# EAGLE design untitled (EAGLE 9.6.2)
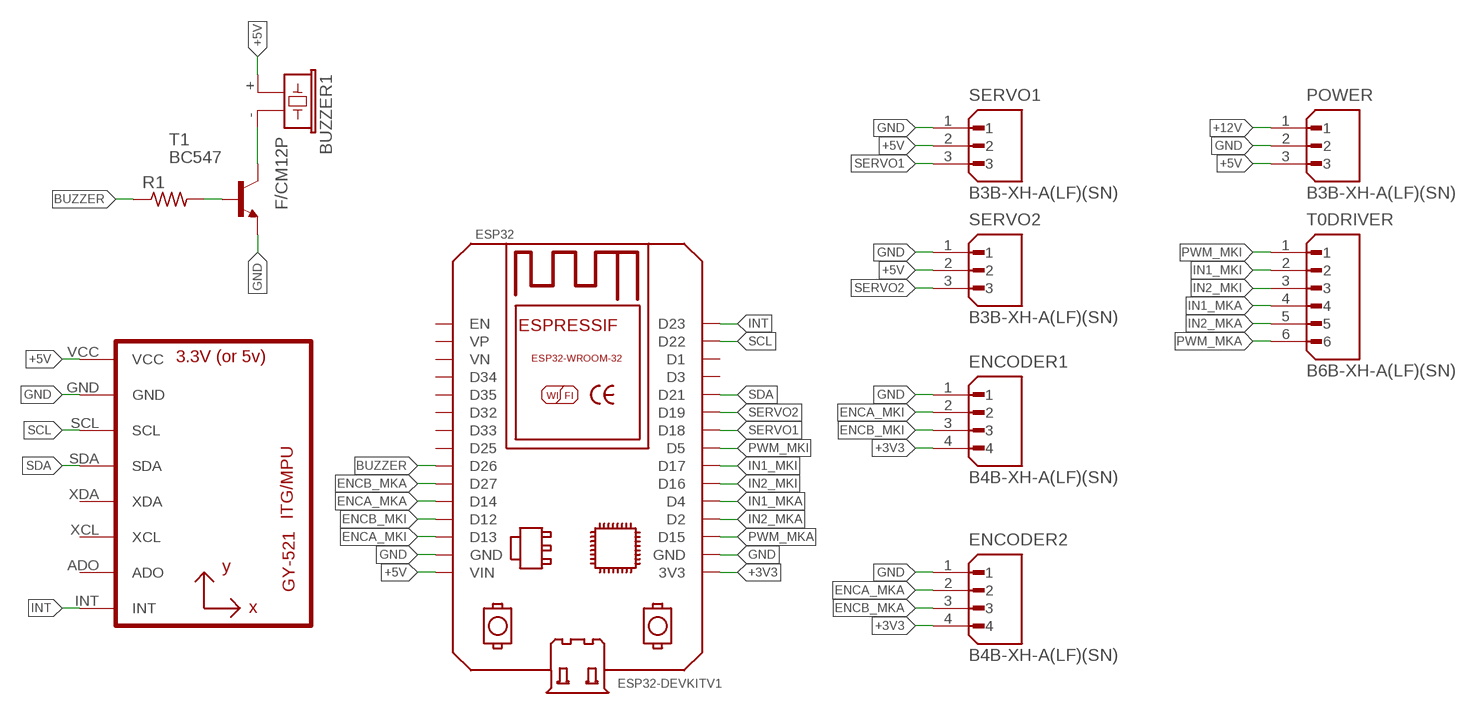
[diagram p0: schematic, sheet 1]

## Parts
BUZZER1  F/CM12P  [F/CM12P]
ENCODER1  B4B-XH-A(LF)(SN)  [JST_B4B-XH-A(LF)(SN)]
ENCODER2  B4B-XH-A(LF)(SN)  [JST_B4B-XH-A(LF)(SN)]
ESP32  ESP32DEVKITV1  [ESP32-DEVKITV1]
POWER  B3B-XH-A(LF)(SN)  [JST_B3B-XH-A(LF)(SN)]
R1  R-US_0204/7  [0204/7]
SERVO1  B3B-XH-A(LF)(SN)  [JST_B3B-XH-A(LF)(SN)]
SERVO2  B3B-XH-A(LF)(SN)  [JST_B3B-XH-A(LF)(SN)]
T0DRIVER  B6B-XH-A(LF)(SN)  [JST_B6B-XH-A(LF)(SN)]
T1  BC547  [TO92]
U2  GY-521MPU6050  [GY-521]

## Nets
+3V3: ENCODER1.4 ENCODER2.4 ESP32.3V3
+5V: BUZZER1.+ ESP32.VIN POWER.3 SERVO1.2 SERVO2.2 U2.VCC
+12V: POWER.1
BUZZER: ESP32.D26 R1.1
ENCA_MKA: ENCODER2.2 ESP32.D14
ENCA_MKI: ENCODER1.2 ESP32.D13
ENCB_MKA: ENCODER2.3 ESP32.D27
ENCB_MKI: ENCODER1.3 ESP32.D12
GND: ENCODER1.1 ENCODER2.1 ESP32.GND ESP32.GND@1(GND) POWER.2 SERVO1.1 SERVO2.1 T1.1(E) U2.GND
IN1_MKA: ESP32.D4 T0DRIVER.4
IN1_MKI: ESP32.D17 T0DRIVER.2
IN2_MKA: ESP32.D2 T0DRIVER.5
IN2_MKI: ESP32.D16 T0DRIVER.3
INT: ESP32.D23 U2.INT
N$9: BUZZER1.- T1.3(C)
N$10: R1.2 T1.2(B)
PWM_MKA: ESP32.D15 T0DRIVER.6
PWM_MKI: ESP32.D5 T0DRIVER.1
SCL: ESP32.D22 U2.SCL
SDA: ESP32.D21 U2.SDA
SERVO1: ESP32.D18 SERVO1.3
SERVO2: ESP32.D19 SERVO2.3
Unconnected: ESP32.D1 ESP32.D3 ESP32.D25 ESP32.D32 ESP32.D33 ESP32.D34 ESP32.D35 ESP32.EN ESP32.VN ESP32.VP U2.ADO U2.XCL U2.XDA

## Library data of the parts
BUZZER1 = buzzer:F/CM12P: BUZZER; OC_FARNELL: unknown; OC_NEWARK: unknown
ENCODER1 ENCODER2 = JST_4P:B4B-XH-A(LF)(SN): Check availability; AVAILABILITY: In Stock; CHECK_PRICES: https://www.snapeda.com/parts/B4B-XH-A%20%20(LF)(SN)/JST/view-part/?ref=eda; DESCRIPTION: HEADER, VERTICAL, 4WAY; Pitch Spacing: 2.5mm; No. of Contacts: 4Contacts; Gender: Header; Product Range: XH Series; Contact Termination Type: Through Hole; No. of Rows: 1Rows; Contact Plating: Tin Plated Contacts; Contact Material: Brass; SVHC: No SVHC (17-Dec-2015); Contact Resistance: 10mohm; Current Rating: 3A; Insulation Resistance: 1000Mohm; Operating Temperature Max: 85°C; Operating Temperature Min: -25°C; Voltage Rating VAC: 250V; Wire Size AWG Max: 22AWG; Wire Size AWG Min: 30AWG; Withstand Voltage: 1000V; MF: JST; MP: B4B-XH-A (LF)(SN); PACKAGE: None; PRICE: None; SNAPEDA_LINK: https://www.snapeda.com/parts/B4B-XH-A%20%20(LF)(SN)/JST/view-part/?ref=snap
ESP32 = ESP32-DEVKITV1:ESP32DEVKITV1: https://github.com/shridattdudhat
POWER SERVO1 SERVO2 = JST_3P:B3B-XH-A(LF)(SN): Check availability; AVAILABILITY: In Stock; CHECK_PRICES: https://www.snapeda.com/parts/B3B-XH-A%20(LF)(SN)/JST+Sales+America+Inc./view-part/?ref=eda; DESCRIPTION: Connector Header Through Hole 3 position 0.098 (2.50mm); MF: JST Sales America Inc.; MP: B3B-XH-A (LF)(SN); PACKAGE: None; PRICE: None; SNAPEDA_LINK: https://www.snapeda.com/parts/B3B-XH-A%20(LF)(SN)/JST+Sales+America+Inc./view-part/?ref=snap
R1 = rcl:R-US_: RESISTOR, American symbol; SPICEPREFIX: R
T0DRIVER = JST_6P:B6B-XH-A(LF)(SN): Check availability; AVAILABILITY: In Stock; CHECK_PRICES: https://www.snapeda.com/parts/B6B-XH-A(LF)(SN)/JST+Sales+America+Inc./view-part/?ref=eda; DESCRIPTION: Connector Header Through Hole 6 position 0.098 (2.50mm); MF: JST Sales; MP: B6B-XH-A(LF)(SN); PACKAGE: None; PRICE: None; SNAPEDA_LINK: https://www.snapeda.com/parts/B6B-XH-A(LF)(SN)/JST+Sales+America+Inc./view-part/?ref=snap
T1 = transistor:BC547: NPN TRANSISTOR
U2 = gy-521:GY-521

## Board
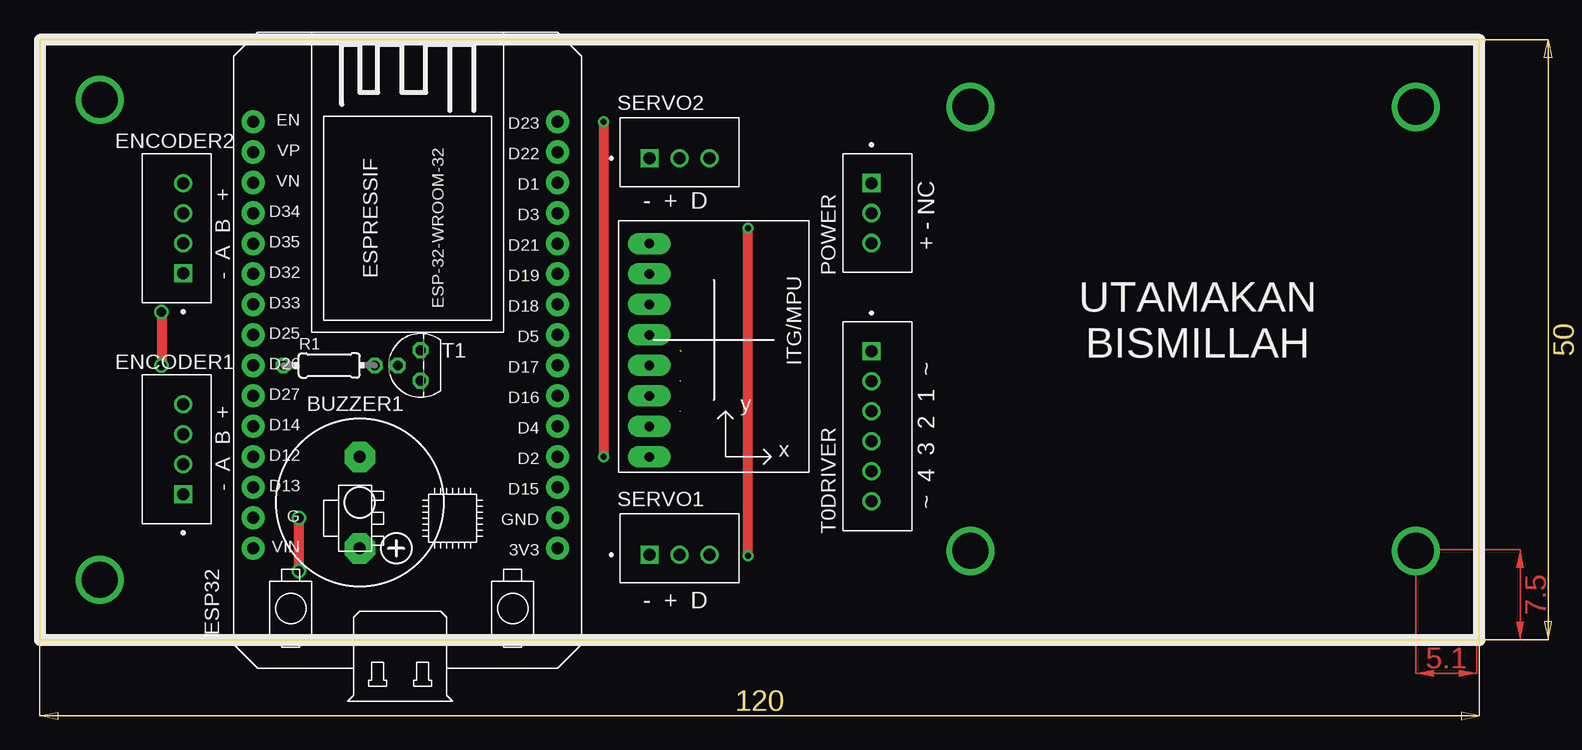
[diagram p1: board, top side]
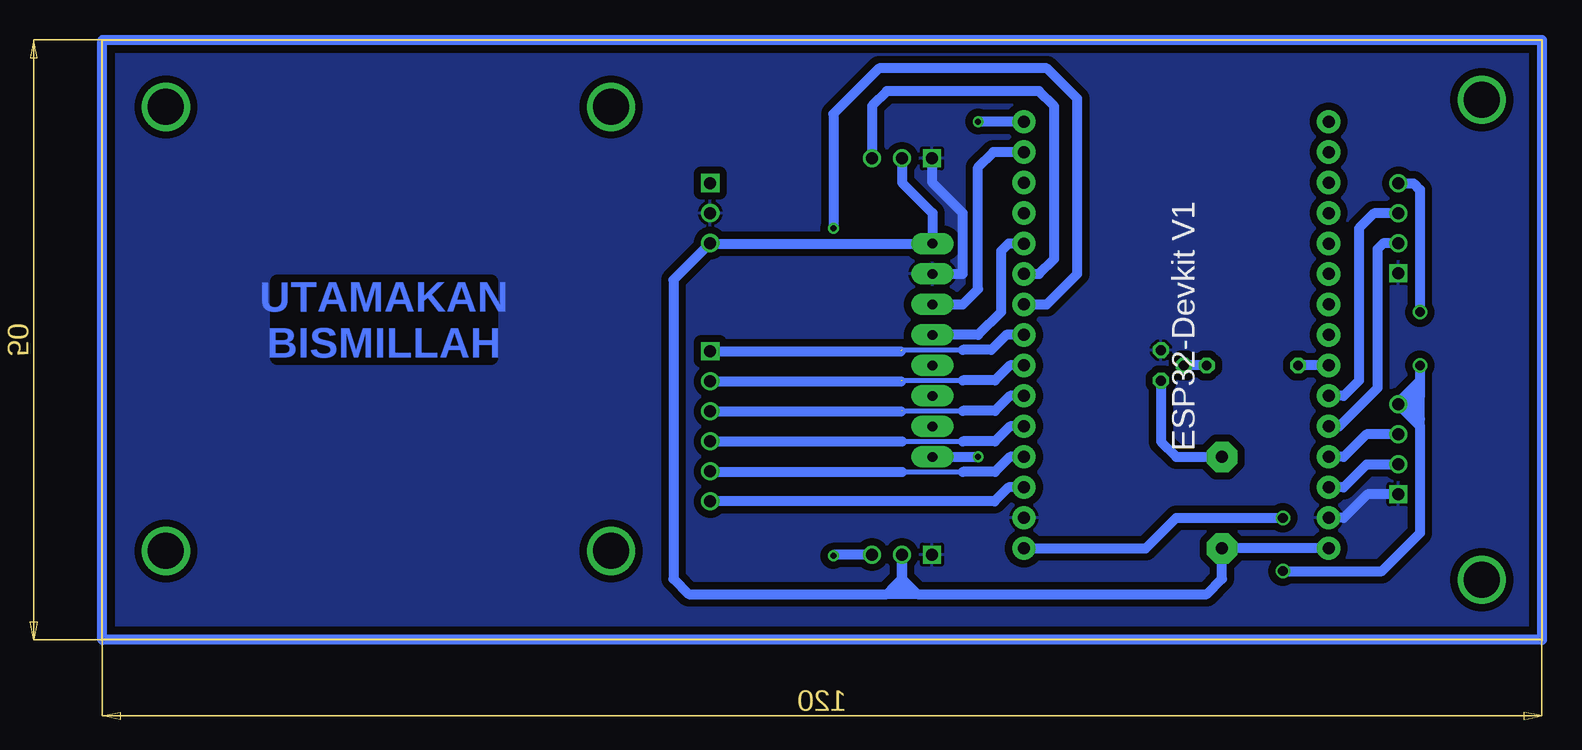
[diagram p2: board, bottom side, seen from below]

Size 126.03 x 56.65 mm. Coordinates in mm from the lower left corner, seen from the top.
Outline: 0,56.65 0,6.65 120,6.65 120,56.65 0,56.65
Copper layers (1*16): Top 0.035mm / dielectric 1.5mm / Bottom 0.035mm
Design rules "default": minimum track width 6mil, minimum drill 0.35mm, track to track 6mil, track to pad 6mil, pad to pad 6mil, via to via 6mil, smd to smd 6mil, copper to edge 40mil, drill to drill 6mil, minimum pad ring 10mil, minimum via ring 8mil, stop-mask expansion 4mil, vias tented up to drill 0mil, thermal gap 10mil

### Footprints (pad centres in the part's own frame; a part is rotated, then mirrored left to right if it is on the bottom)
F/CM12P = drill 1.016 pad 2.54 octagon: + 3.81,0; - -3.81,0
JST_B4B-XH-A(LF)(SN) = drill 1 square: 1 -3.75,-0.525 | drill 1: 2 -1.25,-0.525; 3 1.25,-0.525; 4 3.75,-0.525
ESP32-DEVKITV1 = drill 1 pad 1.93: 3V3 0,0; D1 30.48,0; D2 7.62,0; D3 27.94,0; D4 10.16,0; D5 17.78,0; D12 7.62,25.4; D13 5.08,25.4; D14 10.16,25.4; D15 5.08,0; D16 12.7,0; D17 15.24,0; D18 20.32,0; D19 22.86,0; D21 25.4,0; D22 33.02,0; D23 35.56,0; D25 17.78,25.4; D26 15.24,25.4; D27 12.7,25.4; D32 22.86,25.4; D33 20.32,25.4; D34 27.94,25.4; D35 25.4,25.4; EN 35.56,25.4; GND 2.54,25.4; GND@1 2.54,0; VIN 0,25.4; VN 30.48,25.4; VP 33.02,25.4
JST_B3B-XH-A(LF)(SN) = drill 1 square: 1 -2.5,-0.525 | drill 1: 2 0,-0.525; 3 2.5,-0.525
0204/7 = drill 0.813 octagon: 1 -3.81,0; 2 3.81,0
JST_B6B-XH-A(LF)(SN) = drill 1 square: 1 -6.25,-0.525 | drill 1: 2 -3.75,-0.525; 3 -1.25,-0.525; 4 1.25,-0.525; 5 3.75,-0.525; 6 6.25,-0.525
TO92 = drill 0.813 octagon: 1 1.27,0; 2 0,1.905; 3 -1.27,0
GY-521 = drill 0.8 pad 1.778 long: ADO -8.89,-6.35; GND -8.89,6.35; INT -8.89,-8.89; SCL -8.89,3.81; SDA -8.89,1.27; VCC -8.89,8.89; XCL -8.89,-3.81; XDA -8.89,-1.27

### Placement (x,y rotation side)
BUZZER1  26.67,18.08 270 top
ENCODER1  11.43,22.52 90 top
ENCODER2  11.43,40.94 90 top
ESP32  43.18,14.27 90 top
POWER  69.85,42.21 270 top
R1  24.13,29.51 0 top
SERVO1  53.34,14.27 0 top
SERVO2  53.34,47.29 0 top
T0DRIVER  69.85,24.43 270 top
T1  31.75,29.51 90 top
U2  59.69,30.78 0 top

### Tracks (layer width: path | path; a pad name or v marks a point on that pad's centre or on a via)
+3V3  (via drill 0.8)
  Top 0.813: v21.59,16.81 v21.59,12.36 | v10.16,33.95 v10.16,29.51
  Bottom 0.152: 11.43,26.27 10.86,26.27 10.16,26.97
  Bottom 0.813: ENCODER2.4 10.69,44.69 10.16,44.16 v10.16,33.95 | ESP32.3V3 33.02,14.27 30.48,16.81 v21.59,16.81 | v21.59,12.36 13.34,12.36 10.16,15.54 10.16,24.43 | ENCODER1.4 10.16,24.48 | 10.16,24.48 10.16,25.06 | 10.16,25.06 10.16,26.97 | v10.16,29.51 10.16,28.24 | 10.16,28.24 10.16,28.07 | 10.16,28.07 10.16,26.97 | 10.16,24.48 10.16,24.43 | ENCODER1.4 10.16,28.07 | ENCODER1.4 11.96,26.45 10.16,28.24 | ENCODER1.4 11.96,26.22 10.16,24.43 | ENCODER1.4 11.43,26.27 10.22,26.27 | ENCODER1.4 11.26,26.97 10.16,26.97 | ENCODER1.4 11.37,26.27 10.16,25.06
+5V
  Bottom 0.813: SERVO2.2 53.34,44.75 50.8,42.21 U2.VCC 69.28,39.67 POWER.3 72.39,36.65 72.39,11.73 71.12,10.46 54.61,10.46 | 53.34,11.73 SERVO1.2 53.34,11.2 | 53.34,11.73 52.7,11.09 | 52.7,11.09 52.07,10.46 | 52.07,10.46 27.94,10.46 26.67,11.73 BUZZER1.+ ESP32.VIN | 53.34,11.73 53.98,11.09 | 53.34,10.46 54.61,10.46 | 52.07,10.46 53.34,10.46 | 53.34,10.46 53.98,11.09 | 54.61,10.46 53.98,11.09 | 53.98,11.09 52.7,11.09
BUZZER
  Bottom 0.813: ESP32.D26 R1.1
ENCA_MKA
  Bottom 0.813: ESP32.D14 16.89,24.43 13.72,27.61 13.72,39.2 13.22,39.69 ENCODER2.2
ENCA_MKI
  Bottom 0.813: ENCODER1.2 11.97,21.25 14.61,21.25 16.51,19.35 ESP32.D13
ENCB_MKA
  Bottom 0.813: ESP32.D27 16.51,26.97 15.24,28.24 15.24,40.94 13.99,42.19 ENCODER2.3
ENCB_MKI
  Bottom 0.813: ENCODER1.3 14.62,23.77 16.51,21.89 ESP32.D12
GND
  Bottom 0.813: ESP32.GND 16.51,16.81 14.54,18.77 ENCODER1.1 11.89,18.71 | SERVO2.1 50.84,44.79 48.26,42.21 48.26,37.13 U2.GND
  pour Bottom (isolate 0.61): 0,6.65 120,6.65 120,56.65 0,56.65
IN1_MKA
  Bottom 0.406: 53.34,23.18 48.26,23.18
  Bottom 0.813: ESP32.D4 44.34,24.43 45.59,23.18 48.26,23.18 | T0DRIVER.4 53.34,23.18
IN1_MKI  (1 unrouted)
  Bottom 0.406: 53.34,28.26 48.26,28.26
  Bottom 0.813: ESP32.D17 44.34,29.51 45.59,28.26 48.26,28.26 | T0DRIVER.2 53.42,28.18
IN2_MKA
  Bottom 0.406: 53.34,20.64 48.26,20.64
  Bottom 0.813: ESP32.D2 44.34,21.89 45.59,20.64 48.26,20.64 | T0DRIVER.5 69.29,20.64 53.34,20.64
IN2_MKI  (1 unrouted)
  Bottom 0.406: 53.34,25.72 48.26,25.72
  Bottom 0.813: ESP32.D16 44.34,26.97 45.59,25.72 48.26,25.72 | T0DRIVER.3 53.38,25.68
INT  (via drill 0.5)
  Top 0.813: v46.99,49.83 v46.99,21.89
  Bottom 0.813: ESP32.D23 v46.99,49.83 | U2.INT v46.99,21.89
N$1
  Bottom 0.813: 0,6.65 120,6.65 120,56.65 0,56.65 0,6.65
N$9
  Bottom 0.813: T1.3 31.75,23.16 30.48,21.89 BUZZER1.-
N$10
  Bottom 0.813: R1.2 T1.2
N$11  (via drill 3)
  other vias: 5,51.65
N$12  (via drill 3)
  other vias: 5,11.65
N$13  (via drill 3)
  other vias: 77.59,14.05
N$14  (via drill 3)
  other vias: 77.59,51.05
N$15  (via drill 3)
  other vias: 114.7,51.05
N$16  (via drill 3)
  other vias: 114.7,14.05
PWM_MKA
  Bottom 0.813: ESP32.D15 44.45,19.35 45.62,18.18 T0DRIVER.6
PWM_MKI  (1 unrouted)
  Bottom 0.406: 53.34,30.8 48.26,30.8
  Bottom 0.813: ESP32.D5 44.64,32.05 45.89,30.8 48.26,30.8 | T0DRIVER.1 53.47,30.68
SCL
  Bottom 0.813: U2.SCL 48.26,34.59 46.99,35.86 46.99,46.02 45.72,47.29 ESP32.D22
SDA
  Bottom 0.813: ESP32.D21 44.45,39.67 45.09,39.03 45.09,33.95 46.99,32.05 U2.SDA
SERVO1  (via drill 0.5)
  Top 0.813: v59.05,13.63 v59.05,40.94
  Bottom 0.813: ESP32.D18 41.27,34.59 38.73,37.13 38.73,51.73 41.27,54.27 55.24,54.27 59.05,50.46 v59.05,40.94 | SERVO1.3 58.95,13.74 v59.05,13.63
SERVO2
  Bottom 0.813: ESP32.D19 41.91,37.13 40.64,38.4 40.64,51.1 41.91,52.37 54.61,52.37 55.84,51.14 SERVO2.3
(copper drawn outside any net)
  shapes: Top area x2

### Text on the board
Bottom: UTAMAKAN / BISMILLAH
tPlace: - + D | + - NC | - A B + | UTAMAKAN / BISMILLAH | - A B + | ~ 4 3 2 1 ~ | - + D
